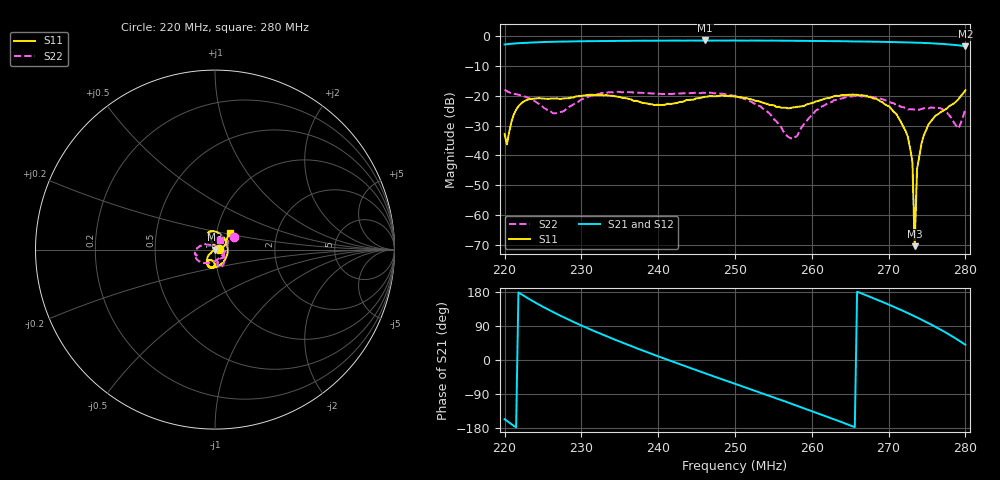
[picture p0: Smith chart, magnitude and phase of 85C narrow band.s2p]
!Agilent Technologies,E8362C,SG49020144,A.09.33.09
!Agilent E8362C: A.09.33.09
!Date: Friday, October 10, 2025 10:00:23
!Correction: S11(Full 2 Port(1,2))
!S21(Full 2 Port(1,2))
!S12(Full 2 Port(1,2))
!S22(Full 2 Port(1,2))
!S2P File: Measurements: S11, S21, S12, S22:
# Hz S  dB  R 50
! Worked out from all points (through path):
!   201 points, 220 MHz to 280 MHz, reference 50 ohm
!   highest |S21| = -1.40 dB at 246.1 MHz (marker M1); lowest = -3.4 dB at 280 MHz (marker M2)
!   lowest |S11| = -70.4 dB at 273.4 MHz (marker M3), VSWR 1.00, Z = 50 - j0.0301 ohm
!   |S11| at or under -10 dB: start of sweep to end of sweep
!   |S22| runs from -34.4 to -17.9 dB; largest |S21 - S12| = 0.0075
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2.2e8  -32.80 3.2  -2.73 -156.3  -2.75 -156.2  -17.90 34.9
2.203e8  -36.27 56.5  -2.66 -160.8  -2.64 -160.9  -18.42 38.2
2.212e8  -26.21 113.0  -2.44 -173.8  -2.41 -173.7  -19.29 44.3
2.227e8  -21.59 110.8  -2.20 167.0  -2.20 166.8  -20.27 42.5
2.266e8  -20.91 110.6  -1.84 123.6  -1.83 123.6  -25.86 -39.8
2.302e8  -19.89 112.5  -1.67 89.3  -1.65 89.4  -20.95 -122.3
2.353e8  -20.62 75.2  -1.53 46.2  -1.53 46.1  -18.80 -158.1
2.401e8  -23.03 3.6  -1.46 8.9  -1.45 9.0  -19.31 -164.0
2.461e8  -20.29 -83.7  -1.40 -35.1  -1.46 -35.1  -19.00 -169.4
2.5e8  -20.21 -112.1  -1.43 -62.8  -1.46 -62.9  -19.98 175.3
2.575e8  -23.89 -104.8  -1.48 -116.4  -1.48 -116.6  -34.40 46.7
2.602e8  -22.30 -91.8  -1.55 -136.4  -1.54 -136.2  -25.91 -26.3
2.656e8  -19.60 -106.0  -1.72 -177.2  -1.72 -177.6  -19.90 -66.7
2.701e8  -23.60 -130.7  -1.88 145.3  -1.94 145.6  -21.92 -80.5
2.728e8  -37.60 -150.0  -2.08 121.1  -2.08 121.0  -24.50 -63.1
2.731e8  -42.05 -138.9  -2.11 118.1  -2.09 118.1  -24.53 -61.0
2.734e8  -70.43 -93.0  -2.13 115.0  -2.12 115.2  -24.57 -57.1
2.737e8  -44.66 22.8  -2.17 112.3  -2.16 112.3  -24.57 -54.9
2.746e8  -33.10 21.7  -2.22 103.5  -2.23 103.2  -24.15 -47.6
2.77e8  -25.13 20.0  -2.55 77.8  -2.55 77.6  -24.43 -38.0
2.791e8  -21.08 41.5  -3.02 52.0  -3.04 52.0  -30.87 15.2
2.8e8  -18.11 49.4  -3.36 40.0  -3.33 39.9  -24.33 63.5
